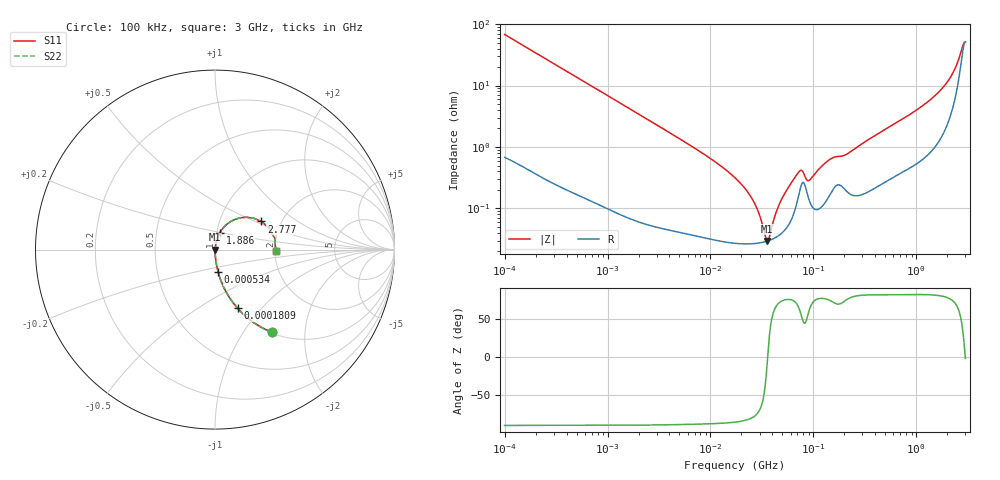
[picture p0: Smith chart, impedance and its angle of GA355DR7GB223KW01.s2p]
!Murata Part Number: GA355DR7GB223KW01
!These Parameters are Measured in Series Mode Connection
!Data Generated on Jun 19, 2026
!  o--ll--o
!Port1  Port2
!  o------o
!Operation Temp=25[degC], DC Bias Voltage=0[V]
!Freq. Start=100[kHz] Stop=3[GHz] 401[Steps]
# Hz S RI R 50
!Freq.(Hz) S11(Real) S11(Imag) S21(Real) S21(Imag) S12(Real) S12(Imag) S22(Real) S22(Imag)
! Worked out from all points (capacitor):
!   401 points, 100 kHz to 3 GHz, reference 50 ohm
!   read as one part in series: C = 23.5 nF near 105.3 kHz
!   lowest |Z| = 29.7 mohm at 35.64 MHz (marker M1)
!   series resonance near 35.92 MHz, so ESL is about 840 pH
!   S11 on the Smith chart (normalised r, x): 100 kHz: 1.01, -1.35; 180.9 kHz: 1.01, -0.75; 534 kHz: 1.00, -0.26; 1.886 GHz: 1.04, +0.20; 2.777 GHz: 1.58, +0.55; 3 GHz: 2.02, -0.03
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100000  0.3156 -0.4598  0.6844 0.4598  0.6844 0.4598  0.3156 -0.4598
180898  0.1263 -0.3269  0.8737 0.3269  0.8737 0.3269  0.1263 -0.3269
533989  0.0177 -0.1256  0.9823 0.1256  0.9823 0.1256  0.0177 -0.1256
562235  0.0161 -0.1196  0.9839 0.1196  0.9839 0.1196  0.0161 -0.1196
3161081  0.000957 -0.0217  0.999 0.0217  0.999 0.0217  0.000957 -0.0217
1.77727e7  0.000279 -0.00302  0.9997 0.00302  0.9997 0.00302  0.000279 -0.00302
2.616047e7  0.00027 -0.00129  0.9997 0.00129  0.9997 0.00129  0.00027 -0.00129
3.564176e7  0.000295 -3.19e-05  0.9997 3.19e-05  0.9997 3.19e-05  0.000295 -3.19e-05
3.752708e7  0.000304 0.000179  0.9997 -0.000179  0.9997 -0.000179  0.000304 0.000179
4.855934e7  0.000389 0.0013  0.9996 -0.0013  0.9996 -0.0013  0.000389 0.0013
6.965816e7  0.0013 0.0034  0.9987 -0.0034  0.9987 -0.0034  0.0013 0.0034
7.525761e7  0.00223 0.00352  0.9978 -0.00352  0.9978 -0.00352  0.00223 0.00352
8.784301e7  0.00167 0.00229  0.9983 -0.00229  0.9983 -0.00229  0.00167 0.00229
9.738194e7  0.00107 0.00305  0.9989 -0.00305  0.9989 -0.00305  0.00107 0.00305
1.43341e8  0.00166 0.00599  0.9983 -0.00599  0.9983 -0.00599  0.00166 0.00599
2.109903e8  0.00195 0.00738  0.9981 -0.00738  0.9981 -0.00738  0.00195 0.00738
5.475153e8  0.00337 0.0208  0.9966 -0.0208  0.9966 -0.0208  0.00337 0.0208
1.186261e9  0.00877 0.0475  0.9912 -0.0475  0.9912 -0.0475  0.00877 0.0475
1.886474e9  0.0272 0.0943  0.9728 -0.0943  0.9728 -0.0943  0.0272 0.0943
2.378954e9  0.0835 0.154  0.9165 -0.154  0.9165 -0.154  0.0835 0.154
2.776789e9  0.2582 0.1571  0.7418 -0.1571  0.7418 -0.1571  0.2582 0.1571
3e9  0.3387 -0.00586  0.6613 0.00586  0.6613 0.00586  0.3387 -0.00586
